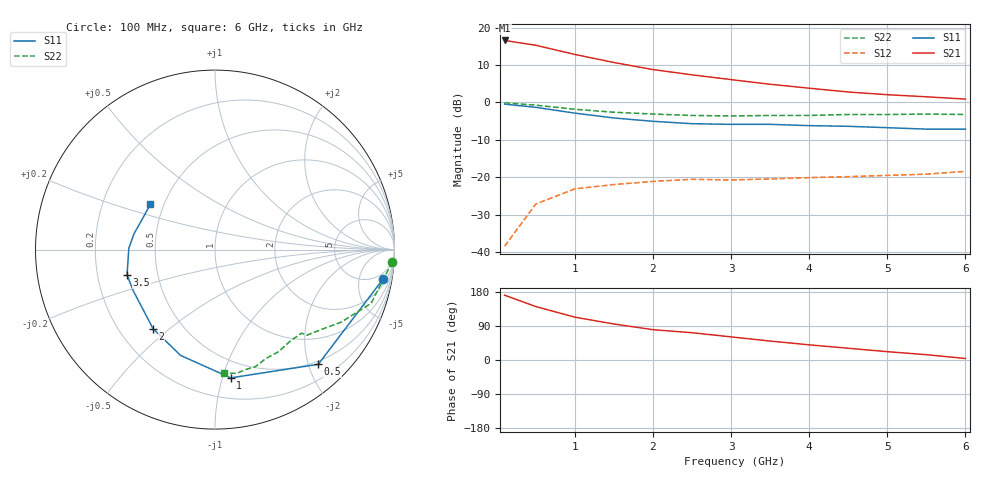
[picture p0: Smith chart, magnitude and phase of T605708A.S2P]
!AT-60570
!S-PARAMETERS at Vce=8V  Ic=2mA.  LAST UPDATED 07-21-92
# ghz s ma r 50
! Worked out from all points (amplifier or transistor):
!   13 points, 100 MHz to 6 GHz, reference 50 ohm
!   highest |S21| = 16.6 dB at 100 MHz (marker M1)
!   |S21| within 3 dB of that: start of sweep to 848.5 MHz
!   unconditionally stable (mu >= 1): 2.73 GHz to end of sweep
!   at 1 GHz: K = 0.43, MSG = 18.0 dB, |S12| = -23.1 dB
!   at 3 GHz: K = 1.09, MAG = 11.6 dB, |S12| = -20.7 dB
!   at 6 GHz: K = 1.40, MAG = 5.9 dB, |S12| = -18.4 dB
!   lowest NFmin = 1.40 dB at 1 GHz
!   S11 on the Smith chart (normalised r, x): 100 MHz: 3, -11; 500 MHz: 0.44, -2.17; 1 GHz: 0.36, -1.06; 2 GHz: 0.34, -0.44; 3.5 GHz: 0.33, -0.13; 6 GHz: 0.42, +0.26
0.1  0.95 -10.0  6.74 171.0  0.012 86.0  0.99 -4.0
0.5  0.86 -48.0  5.81 141.0  0.044 63.0  0.92 -19.0
1  0.72 -83.0  4.38 113.0  0.07 43.0  0.81 -30.0
1.5  0.62 -108.0  3.42 95.0  0.08 35.0  0.74 -37.0
2  0.56 -128.0  2.75 80.0  0.088 28.0  0.7 -43.0
2.5  0.52 -141.0  2.34 72.0  0.094 28.0  0.67 -44.0
3  0.51 -153.0  2.02 61.0  0.092 27.0  0.66 -51.0
3.5  0.51 -164.0  1.75 50.0  0.095 24.0  0.67 -58.0
4  0.49 -172.0  1.55 40.0  0.099 25.0  0.67 -65.0
4.5  0.48 179.0  1.38 31.0  0.102 22.0  0.69 -71.0
5  0.46 169.0  1.27 22.0  0.106 21.0  0.69 -76.0
5.5  0.44 158.0  1.19 14.0  0.11 22.0  0.7 -80.0
6  0.44 145.0  1.11 4.0  0.12 20.0  0.69 -86.0
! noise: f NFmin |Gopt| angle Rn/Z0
1  1.4  0.54  48  0.2
2  1.8  0.44  98  0.28
4  2.8  0.4  180  0.28
